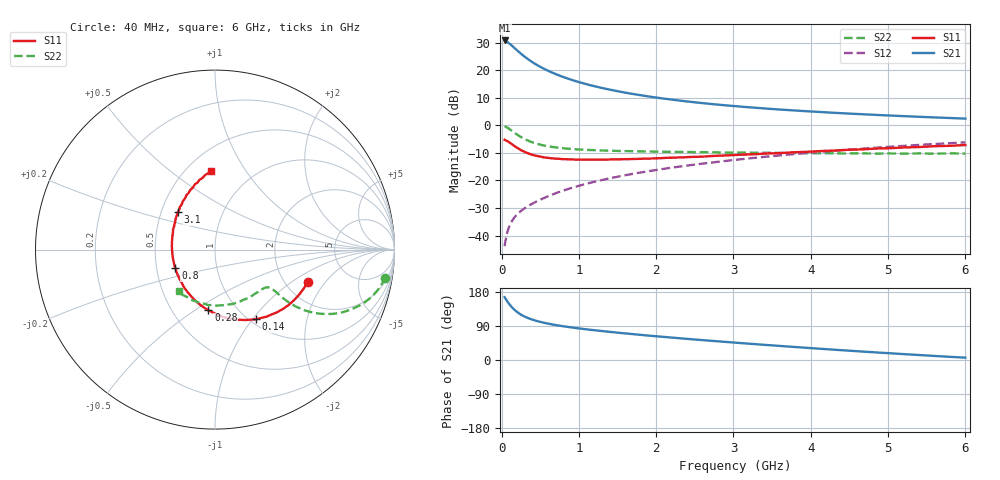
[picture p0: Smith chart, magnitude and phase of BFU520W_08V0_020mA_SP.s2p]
! Filename:  P:\Prog\Test\Noise\ATS_data\Testdata_Net\Run2\BFU520W_APM2013_06_A05_08p0V_020mA_SP_CM01_D.s2p
! Date/Time: Tue 26/Mar/2013 18:01:43
! BFU520W_APM2013_06_A05_08p0V_1to20mA_SP_CM01_Bias8_R.s2p
! MDIF S-parameter v. bias file
! BFU520W_APM2013_06_A05_08p0V_1to20mA_SP_CM01
! Date/time Thu Mar 21 15:28:29 2013
! VAR V_out= 8.0000
! VAR I_out= 19.9950
! VAR V_in= 0.8195
! VAR I_in= 0.2204
! Device data file deembeded for feedlines and parallel
! Original file: \Run2\BFU520W_APM2013_06_A05_08p0V_020mA_SP_CM01_R.s2p
! Feed-files: PR019V01_070313_Feed1.s2p, PR019V01_070313_Feed2.s2p
! Parallel-file: PR019V01_070313_Par.s2p
# MHz S MA R 50
!  Freq-MHz  S11-mag  S11-arg  S21-mag  S21-arg  S12-mag  S12-arg  S22-mag  S22-arg
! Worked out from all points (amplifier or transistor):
!   98 points, 40 MHz to 6 GHz, reference 50 ohm
!   highest |S21| = 30.8 dB at 40 MHz (marker M1)
!   |S21| within 3 dB of that: start of sweep to 177.8 MHz
!   unconditionally stable (mu >= 1): 1.108 GHz to 2.184 GHz
!   at 300 MHz: K = 0.69, MSG = 27.5 dB, |S12| = -30.1 dB
!   at 1.6 GHz: K = 1.01, MAG = 14.3 dB, |S12| = -18.1 dB
!   at 6 GHz: K = 0.87, MSG = 4.3 dB, |S12| = -6.2 dB
!   S11 on the Smith chart (normalised r, x): 40 MHz: 2.65, -1.35; 140 MHz: 1.07, -1.04; 280 MHz: 0.74, -0.57; 800 MHz: 0.63, -0.14; 3.1 GHz: 0.61, +0.28; 6 GHz: 0.65, +0.71
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40  0.547 -19.0  34.75 165.7  0.006432 82.2  0.9622 -9.3
50  0.54 -23.6  34.46 162.4  0.007896 80.8  0.9496 -11.5
60  0.5318 -28.1  33.51 159.2  0.0094 79.3  0.936 -13.8
90  0.503 -41.0  31.43 150.3  0.01339 75.2  0.8836 -19.5
120  0.4707 -52.6  29.13 142.5  0.01684 72.0  0.8254 -24.0
140  0.4499 -59.5  27.5 138.0  0.01887 70.5  0.7869 -26.5
160  0.4293 -66.1  25.91 133.9  0.02082 69.2  0.7504 -28.5
200  0.3936 -77.6  23.05 127.0  0.02415 67.7  0.6843 -31.4
240  0.3636 -87.6  20.62 121.2  0.02715 67.0  0.6294 -33.4
280  0.3396 -96.3  18.53 116.6  0.02998 66.8  0.5842 -34.5
320  0.3207 -104.0  16.78 112.7  0.03273 67.0  0.5475 -35.2
360  0.3055 -110.7  15.28 109.4  0.03541 67.3  0.5176 -35.5
460  0.2788 -124.7  12.44 102.8  0.0421 68.4  0.4635 -35.5
600  0.2578 -139.5  9.838 96.1  0.05165 70.0  0.4177 -34.9
800  0.2438 -154.9  7.535 89.0  0.06568 71.3  0.3845 -34.8
1050  0.2392 -168.9  5.838 82.2  0.08368 72.0  0.3626 -35.5
1500  0.2414 173.1  4.173 72.1  0.117 71.6  0.3444 -39.5
2050  0.2535 157.2  3.126 61.8  0.1589 69.5  0.3339 -46.5
3100  0.2937 134.6  2.186 44.6  0.2434 63.3  0.3212 -64.3
4100  0.3406 118.2  1.756 30.0  0.3288 55.7  0.3115 -84.8
5200  0.3974 102.7  1.472 15.6  0.4248 45.8  0.3068 -110.2
6000  0.4402 92.5  1.326 6.2  0.4919 37.9  0.3079 -130.9
